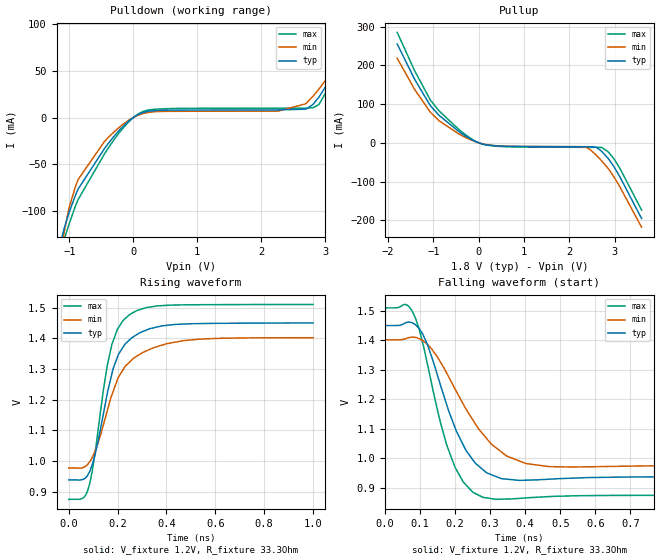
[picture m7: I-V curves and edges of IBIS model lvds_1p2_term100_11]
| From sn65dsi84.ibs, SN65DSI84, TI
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|   Model
[Model]   lvds_1p2_term100_11
Model_type   Output
Polarity   Non-Inverting
Vmeas = 1.2
Vref = 1.2
Cref = 1pF
Rref = 50
|   typ   min   max
C_comp   0.4797pF   0.3035pF   0.7186pF
[Voltage Range]   1.8   1.65   1.95
[Temperature Range]   27   125   -40
[Pullup Reference]   1.8   1.65   1.95
[Pulldown Reference]   -0   -0   -0
[Power Clamp Reference]   1.8   1.65   1.95
[GND Clamp Reference]   -0   -0   -0
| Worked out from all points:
|   slope of the pulldown table from 0 to 0.27 V, typ, clamps not added: 38.9 ohm
|   slope of the pullup table from 0 to 0.27 V, typ, clamps not added: 40.4 ohm
|   falling waveform, V_fixture 1.2V, R_fixture 33.3Ohm: 20-80 % time 93.3ps typ, 131ps min, 80.5ps max; typ from 1.45 V to 0.938 V
|   rising waveform, V_fixture 1.2V, R_fixture 33.3Ohm: 20-80 % time 90ps typ, 121ps min, 75ps max; typ from 0.938 V to 1.45 V
[Pulldown]
|   Voltage   I(typ)   I(min)   I(max)
-1.8V     -664mA     -698.6mA   -654.8mA
-1.103V   -124.3mA   -132.7mA   -135.5mA
-1.076V   -117.1mA   -120.7mA   -129.1mA
-1.006V   -101.7mA   -96.58mA   -113.9mA
-860.4mV  -75.94mA   -65.77mA   -87.07mA
-374.4mV  -26.16mA   -20.13mA   -30.86mA
-88.2mV   -4.783mA   -3.651mA   -5.747mA
144mV     5.138mA    4.059mA    6.205mA
2.261V    8.081mA    6.81mA     9.947mA
2.698V    8.92mA     14.75mA    10.01mA
2.898V    21.48mA    30.03mA    13.71mA
3.595V    96.24mA    93.34mA    94.7mA
[Pullup]
|   Voltage   I(typ)   I(min)   I(max)
-1.8V     254.9mA    218.1mA    285.1mA
-1.406V   162.1mA    136.2mA    184mA
-1.06V    94.68mA    77.94mA    109.2mA
-860.4mV  69.36mA    55.51mA    80.51mA
-250.2mV  14.49mA    11.44mA    17.28mA
9mV       -371.1uA   -314.1uA   -424.9uA
306mV     -7.121mA   -6.823mA   -7.97mA
2.374V    -10.12mA   -11.61mA   -11.72mA
2.596V    -11.67mA   -32.21mA   -11.8mA
2.876V    -43.2mA    -69.27mA   -25.79mA
3.109V    -86.33mA   -112.2mA   -64.5mA
3.595V    -195.3mA   -217.7mA   -173.3mA
[Ramp]
R_load = 33.3
|   typ   min   max
dV/dt_r   0.307022/8.99673e-11   0.254829/1.20605e-10   0.381065/7.50125e-11
dV/dt_f   0.307388/9.32851e-11   0.254829/1.30805e-10   0.381071/8.04559e-11
[Falling Waveform]
V_fixture = 1.2V
V_fixture_min = 1.2V
V_fixture_max = 1.2V
R_fixture = 33.3Ohm
C_fixture = 0F
|   Time   V(typ)   V(min)   V(max)
0s        1.45V      1.402V     1.51V
58.42ps   1.459V     1.406V     1.522V
78.53ps   1.459V     1.411V     1.497V
121ps     1.386V     1.386V     1.32V
176.4ps   1.181V     1.288V     1.044V
222.8ps   1.047V     1.185V     920.9mV
251.1ps   994.6mV    1.13V      885.1mV
303.1ps   945.2mV    1.049V     863.9mV
401.1ps   926.3mV    983mV      866.2mV
1ns       937.9mV    977.2mV    875mV
[Rising Waveform]
V_fixture = 1.2V
V_fixture_min = 1.2V
V_fixture_max = 1.2V
R_fixture = 33.3Ohm
C_fixture = 0F
|   Time   V(typ)   V(min)   V(max)
0s        938.4mV    977.2mV    875.1mV
58.42ps   940.1mV    978.6mV    879.2mV
78.53ps   955mV      989.9mV    905.8mV
107.7ps   1.021V     1.032V     1.027V
141.6ps   1.153V     1.117V     1.231V
176.4ps   1.284V     1.215V     1.38V
203.4ps   1.348V     1.273V     1.435V
251.1ps   1.397V     1.324V     1.479V
467.7ps   1.446V     1.392V     1.509V
1ns       1.45V      1.402V     1.51V
